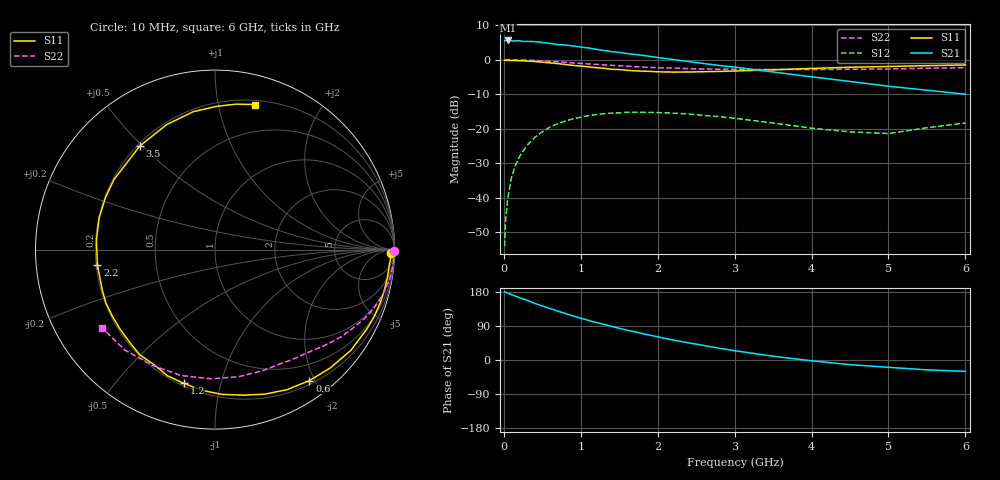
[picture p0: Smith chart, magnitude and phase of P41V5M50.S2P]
! SIEMENS Small Signal Semiconductors
! BFP182
! Si NPN RF Bipolar Junction Transistor in SOT143
! VCE = 1.5 V  IC = 0.5 mA
! Common Emitter S-Parameters:  March  1996
# GHz  S  MA  R  50
!  f  S11  S21  S12  S22
! GHz  MAG  ANG  MAG  ANG  MAG  ANG  MAG  ANG
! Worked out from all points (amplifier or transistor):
!   36 points, 10 MHz to 6 GHz, reference 50 ohm
!   highest |S21| = 5.6 dB at 50 MHz (marker M1)
!   |S21| within 3 dB of that: start of sweep to 1.33 GHz
!   unconditionally stable (mu >= 1): 2.921 GHz to end of sweep
!   at 250 MHz: K = 0.09, MSG = 15.9 dB, |S12| = -26.4 dB
!   at 1.4 GHz: K = 0.51, MSG = 8.9 dB, |S12| = -15.5 dB
!   at 6 GHz: K = 1.24, MAG = 1.2 dB, |S12| = -18.3 dB
!   S11 on the Smith chart (normalised r, x): 10 MHz: 57, -54; 600 MHz: 0.25, -1.93; 1.2 GHz: 0.21, -0.77; 2.2 GHz: 0.21, -0.06; 3.5 GHz: 0.21, +0.49; 6 GHz: 0.24, +1.29
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0.01  0.9817 -1.0  1.87 179.6  0.002 85.8  0.9989 -0.3
0.02  0.9819 -1.8  1.877 179.2  0.0043 88.7  0.997 -0.6
0.05  0.9755 -4.7  1.897 176.3  0.0098 88.5  0.9982 -1.6
0.1  0.9734 -9.1  1.873 172.5  0.0197 83.3  0.9969 -3.4
0.2  0.9662 -18.6  1.883 164.8  0.0389 77.6  0.9921 -6.9
0.3  0.955 -27.5  1.838 157.8  0.0573 72.0  0.9845 -10.2
0.4  0.9423 -36.6  1.827 149.6  0.0748 66.0  0.9735 -13.5
0.6  0.8997 -54.2  1.721 135.9  0.1057 54.7  0.9465 -19.6
0.8  0.8522 -70.9  1.629 122.7  0.1295 44.5  0.916 -25.0
0.9  0.8255 -79.2  1.582 116.3  0.1394 39.6  0.897 -27.6
1.1  0.7872 -95.5  1.475 104.5  0.1549 31.0  0.867 -32.3
1.2  0.7653 -103.1  1.411 99.3  0.1604 26.3  0.8541 -34.7
1.6  0.7018 -132.7  1.225 78.8  0.1731 12.4  0.8058 -42.3
1.9  0.6767 -153.9  1.115 65.5  0.1722 3.7  0.7732 -47.8
2.2  0.6607 -172.7  1.007 52.8  0.1683 -3.7  0.7537 -53.1
2.8  0.6756 154.6  0.824 31.1  0.1499 -15.2  0.7271 -64.4
3.5  0.7136 125.9  0.663 10.0  0.1213 -21.8  0.7207 -79.6
4  0.7469 111.1  0.565 -2.1  0.1021 -19.5  0.7201 -91.9
4.5  0.7778 99.0  0.484 -12.3  0.0902 -12.5  0.7266 -105.1
5  0.7975 89.6  0.413 -19.3  0.0853 1.9  0.7333 -118.4
5.5  0.8188 81.8  0.362 -26.0  0.1035 9.9  0.752 -132.0
6  0.8381 74.6  0.316 -29.9  0.1214 12.1  0.765 -145.1
